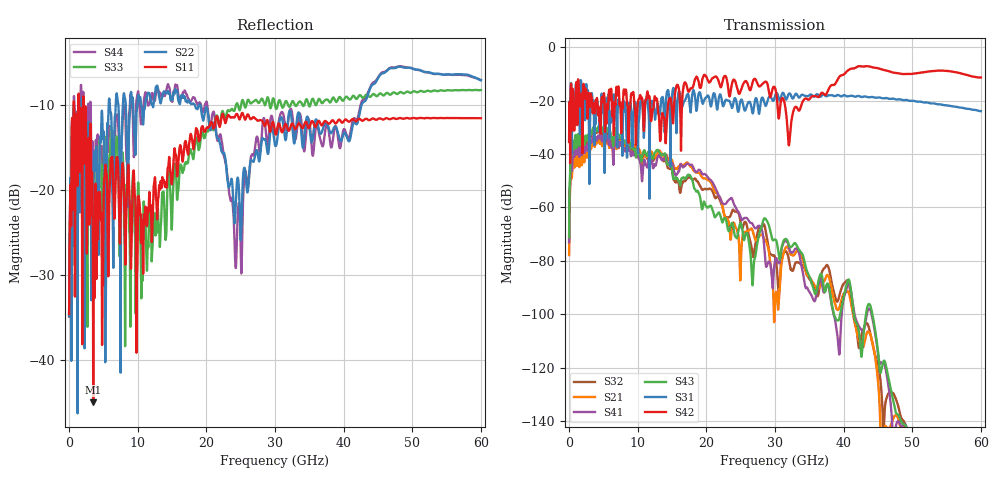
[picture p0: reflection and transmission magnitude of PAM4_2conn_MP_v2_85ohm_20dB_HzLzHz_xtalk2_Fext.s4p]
! Info: Touchstone file created by Circ.  Input file=FAB50GbE_2conn_Midplane_Examax_Topo2_v2_85ohm_20dB_HzLzHz.circ
# Hz S RI R 50
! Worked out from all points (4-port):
!   6000 points, 10 MHz to 60 GHz, reference 50 ohm
!   strongest paths, dB at 10 MHz, 15.01 GHz, 30.01 GHz, 45.01 GHz, 60 GHz:
!     S42: -35.5, -24.0, -15.3, -7.9, -11.4
!     S31: -35.3, -18.0, -18.3, -18.9, -24.0
!     S43: -71.2, -45.8, -72.0, -113.8, -162.2
!     S41: -73.1, -43.4, -80.0, -114.5, -167.5
!     S21: -77.8, -42.4, -94.8, -124.9, -169.6
!     S32: -72.9, -46.1, -78.8, -119.1, -154.8
!   lowest |S11| = -45.0 dB at 3.52 GHz (marker M1), VSWR 1.01, Z = 50.3 - j0.477 ohm
!   |S11| at or under -10 dB: start of sweep to 676.6 MHz; 735.9 MHz to 1.321 GHz (584.8 MHz wide, 56.9 % of centre); 2.144 GHz to end of sweep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
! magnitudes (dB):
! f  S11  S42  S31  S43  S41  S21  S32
! 10 MHz  -34.7  -35.5  -35.3  -71.2  -73.1  -77.8  -72.9
! 770 MHz  -11.6  -30.6  -20.2  -37.7  -41.0  -45.1  -39.3
! 3.52 GHz  -45.0  -22.6  -20.0  -30.1  -33.4  -35.8  -31.4
! 26.77 GHz  -11.5  -12.9  -24.8  -88.1  -66.4  -69.0  -78.3
! 32.06 GHz  -13.0  -36.5  -17.4  -74.3  -75.1  -76.0  -80.1
! 42.09 GHz  -11.7  -7.2  -18.3  -104.8  -103.8  -108.7  -110.2
! 60 GHz  -11.6  -11.4  -24.0  -162.2  -167.5  -169.6  -154.8
